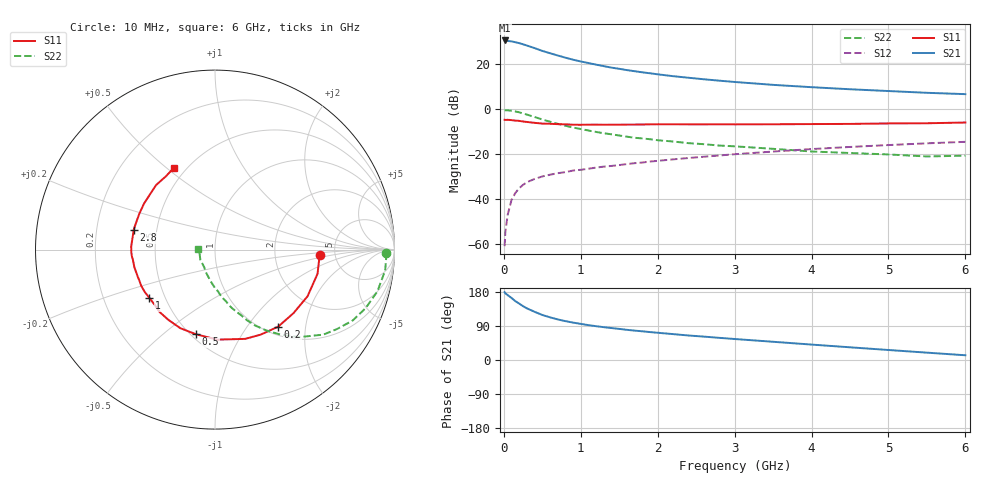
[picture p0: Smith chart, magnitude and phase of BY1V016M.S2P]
! SIEMENS Small Signal Semiconductors
! BFY420
! Si NPN RF SIEGET Grounded Emitter Transistor in MICRO-X
! VCE = 1 V  IC = 16 mA
! Common Emitter S-Parameters:  October  1996
# GHz  S  MA  R  50
!  f  S11  S21  S12  S22
! GHz  MAG  ANG  MAG  ANG  MAG  ANG  MAG  ANG
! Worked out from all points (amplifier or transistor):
!   36 points, 10 MHz to 6 GHz, reference 50 ohm
!   highest |S21| = 30.7 dB at 10 MHz (marker M1)
!   |S21| within 3 dB of that: start of sweep to 363.9 MHz
!   unconditionally stable (mu >= 1): 1.993 GHz to end of sweep
!   at 250 MHz: K = 0.27, MSG = 31.3 dB, |S12| = -33.6 dB
!   at 1.4 GHz: K = 0.89, MSG = 21.9 dB, |S12| = -25.2 dB
!   at 6 GHz: K = 1.10, MAG = 8.7 dB, |S12| = -14.4 dB
!   S11 on the Smith chart (normalised r, x): 10 MHz: 3.80, -0.37; 200 MHz: 1.14, -1.42; 500 MHz: 0.53, -0.65; 1 GHz: 0.41, -0.28; 2.8 GHz: 0.37, +0.10; 6 GHz: 0.43, +0.53
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0.01  0.587 -3.1  34.31 179.0  0.0009 97.3  0.9554 -1.1
0.02  0.583 -5.5  34.26 176.0  0.0019 86.9  0.9552 -2.4
0.1  0.5775 -26.8  32.77 163.7  0.0097 79.2  0.9344 -14.4
0.15  0.5626 -39.0  31.28 155.2  0.0138 73.6  0.9006 -21.2
0.2  0.5551 -50.7  29.91 148.8  0.0176 70.9  0.8625 -27.3
0.25  0.5377 -61.8  28.18 142.0  0.0209 65.1  0.8117 -33.0
0.3  0.5251 -71.3  26.42 136.3  0.0239 63.2  0.7675 -38.1
0.4  0.5018 -88.6  23.16 127.2  0.0283 57.8  0.6758 -46.2
0.5  0.4833 -102.8  20.08 118.8  0.0321 54.7  0.5966 -52.5
0.6  0.4785 -113.9  17.83 112.6  0.0351 53.4  0.5322 -57.7
0.7  0.4698 -123.4  15.89 107.1  0.0379 52.8  0.4788 -62.1
0.8  0.4651 -131.4  14.19 102.6  0.0401 51.2  0.4325 -65.6
1  0.4541 -143.5  11.67 95.3  0.0452 50.8  0.3656 -71.0
1.1  0.4571 -149.1  10.78 92.0  0.0478 51.1  0.3389 -73.9
1.4  0.4563 -161.2  8.515 84.3  0.0551 50.9  0.2788 -80.2
1.6  0.4598 -167.4  7.498 79.6  0.0607 50.7  0.2469 -84.3
2.2  0.4672 177.9  5.495 68.3  0.0771 49.7  0.1926 -94.3
2.8  0.466 166.4  4.366 58.5  0.0941 47.2  0.1567 -103.7
3.5  0.4667 154.6  3.52 48.1  0.1151 43.0  0.1325 -113.7
4.5  0.4754 139.6  2.809 33.5  0.1458 34.8  0.1069 -129.6
5.5  0.4914 123.9  2.342 19.4  0.1757 25.4  0.0895 -162.1
6  0.5106 116.5  2.187 12.5  0.1896 20.4  0.0933 178.9
